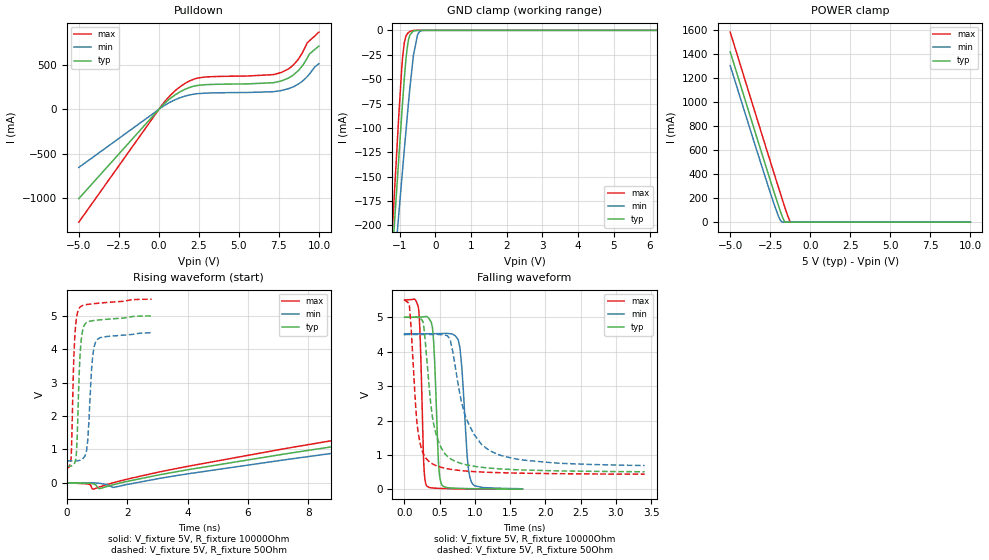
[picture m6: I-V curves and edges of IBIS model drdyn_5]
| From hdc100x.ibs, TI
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|   drdyn_5 Model
[Model]   drdyn_5
Model_type   Open_drain
Polarity   Non-Inverting
Vmeas = 2.5
Vref = 5
Cref = 2pF
Rref = 10000
|   typ   min   max
|   (nom PVT)   (fast PVT)   (slow PVT)
C_comp   1.183e-12   1.138e-12   1.258e-12
| Where nom  PVT is Nominal Process, 5V, 27C
|   Fast PVT is Strong Process,  5.5V, -40C
|   Slow PVT is Weak Process,   4.5V, 150C
[Voltage Range]   5   4.5   5.5
|Junction Temperature
[Temperature Range]   27   150   -40
[Pullup Reference]   5   4.5   5.5
[Pulldown Reference]   0   0   0
[Power Clamp Reference]   5   4.5   5.5
[GND Clamp Reference]   0   0   0
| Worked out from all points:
|   slope of the pulldown table from 0 to 0.75 V, typ, clamps not added: 5.82 ohm
|   GND clamp passes 1 mA (typ) near -0.62 V on its own axis
|   POWER clamp passes 1 mA (typ) near -1.54 V on its own axis
|   falling waveform, V_fixture 5V, R_fixture 10000Ohm: 20-80 % time 56.6ps typ, 80.6ps min, 44.7ps max; typ from 5 V to 0.008 V
|   rising waveform, V_fixture 5V, R_fixture 10000Ohm: 20-80 % time 32.3ns typ, 32.5ns min, 32.4ns max; typ from 0.002 V to 5 V
|   falling waveform, V_fixture 5V, R_fixture 50Ohm: 20-80 % time 176ps typ, 333ps min, 112ps max; typ from 5 V to 0.512 V
|   rising waveform, V_fixture 5V, R_fixture 50Ohm: 20-80 % time 116ps typ, 147ps min, 104ps max; typ from 0.497 V to 4.99 V
[Pulldown]
|   Voltage   I(typ)   I(min)   I(max)
-5V       -1.005A    -654mA     -1.271A
100mV     20.81mA    13.89mA    26.64mA
1.268V    193mA      128.2mA    248.1mA
1.9V      246.6mA    162.6mA    319.7mA
2.5V      272.6mA    179.3mA    356.3mA
7.122V    301.2mA    199.8mA    392.3mA
7.639V    321mA      212.6mA    416.3mA
8.261V    371.5mA    244.9mA    479.4mA
8.734V    442.1mA    288.9mA    571.3mA
9.261V    577.7mA    368.6mA    748.8mA
9.41V     625.6mA    399.5mA    775mA
10V       714.3mA    516.3mA    872.2mA
[GND Clamp]
|   Voltage   I(typ)   I(min)   I(max)
-5V       -1.812A    -1.667A    -1.927A
-1.53V    -409.9mA   -411.7mA   -416.7mA
-1.024V   -131.3mA   -188.2mA   -87.39mA
-940mV    -85.79mA   -152.7mA   -38.51mA
-869.5mV  -49.89mA   -122.8mA   -12.89mA
-825.5mV  -30.72mA   -104.4mA   -6.293mA
-775mV    -14.71mA   -83.7mA    -3.109mA
-715mV    -4.851mA   -59.97mA   -1.221mA
-612.5mV  -598.4uA   -25.38mA   -109.1uA
-500mV    -41.17uA   -4.975mA   -3.075uA
-369.5mV  -1.045uA   -251.8uA   -21.31nA
10V       0A         0A         0A
[POWER Clamp]
|   Voltage   I(typ)   I(min)   I(max)
-5V       1.417A     1.303A     1.582A
-2.732V   447.7mA    342.6mA    606.8mA
-2.043V   160.8mA    69.82mA    314mA
-1.922V   112.2mA    30.38mA    262.8mA
-1.823V   73.97mA    8.2mA      221.4mA
-1.615V   8.322mA    43.69uA    135.5mA
-1.535V   742.4uA    2.928uA    103.1mA
-1.359V   898.3nA    0A         36.17mA
-1.238V   0A         0A         3.593mA
10V       0A         0A         0A
[Ramp]
R_load = 10000
|   typ   min   max
dV/dt_r   2.99835/3.23668e-08   2.71099/3.25143e-08   3.2986/3.24078e-08
dV/dt_f   2.99852/5.6646e-11   2.71117/8.16224e-11   3.29872/4.46603e-11
[Falling Waveform]
V_fixture = 5V
V_fixture_min = 4.5V
V_fixture_max = 5.5V
R_fixture = 10000Ohm
|   Time   V(typ)   V(min)   V(max)
0s        5V         4.5V       5.5V
200.4ps   5.004V     4.522V     5.236V
274.5ps   5.014V     4.522V     699.3mV
312ps     5.023V     4.522V     111.9mV
396.5ps   4.708V     4.523V     41.16mV
483.8ps   718.4mV    4.525V     29.99mV
531.1ps   126.3mV    4.527V     26.36mV
786.9ps   28.83mV    4.116V     14.91mV
947.9ps   20.74mV    222.1mV    11.5mV
1.673ns   8.225mV    17.6mV     6.217mV
[Rising Waveform]
V_fixture = 5V
V_fixture_min = 4.5V
V_fixture_max = 5.5V
R_fixture = 10000Ohm
|   Time   V(typ)   V(min)   V(max)
0s        2.463mV    3.321mV    2.127mV
881.2ps   -31.54mV   1.258mV    -188.2mV
1.542ns   -55.03mV   -137.5mV   5.175mV
9.719ns   1.208V     997.8mV    1.407V
20.71ns   2.468V     2.144V     2.802V
38.9ns    3.808V     3.386V     4.241V
44.7ns    4.5V       3.956V     5.014V
48.78ns   4.755V     4.23V      5.274V
62.32ns   4.969V     4.482V     5.475V
124.2ns   4.997V     4.517V     5.498V
[Falling Waveform]
V_fixture = 5V
V_fixture_min = 4.5V
V_fixture_max = 5.5V
R_fixture = 50Ohm
|   Time   V(typ)   V(min)   V(max)
0s        5V         4.5V       5.5V
71.1ps    5.001V     4.5V       5.29V
175.4ps   5.003V     4.5V       1.972V
260.4ps   4.876V     4.5V       1.067V
364.6ps   2.655V     4.501V     784mV
571.1ps   1.041V     4.482V     615.8mV
648.5ps   896.7mV    4.347V     585.5mV
893.3ps   707.1mV    1.978V     529.3mV
1.209ns   617.5mV    1.121V     494.9mV
3.407ns   511.8mV    692.8mV    440.9mV
[Rising Waveform]
V_fixture = 5V
V_fixture_min = 4.5V
V_fixture_max = 5.5V
R_fixture = 50Ohm
|   Time   V(typ)   V(min)   V(max)
0s        496.7mV    657.5mV    431.7mV
142.9ps   504.7mV    657.5mV    749.7mV
230.4ps   551.9mV    655.6mV    3.642V
293.9ps   699.5mV    655.7mV    4.718V
401.3ps   3.027V     667.3mV    5.206V
476.9ps   4.259V     691.6mV    5.282V
655.4ps   4.796V     958.8mV    5.332V
857.9ps   4.851V     3.783V     5.356V
986.5ps   4.865V     4.266V     5.368V
2.808ns   4.994V     4.49V      5.494V
